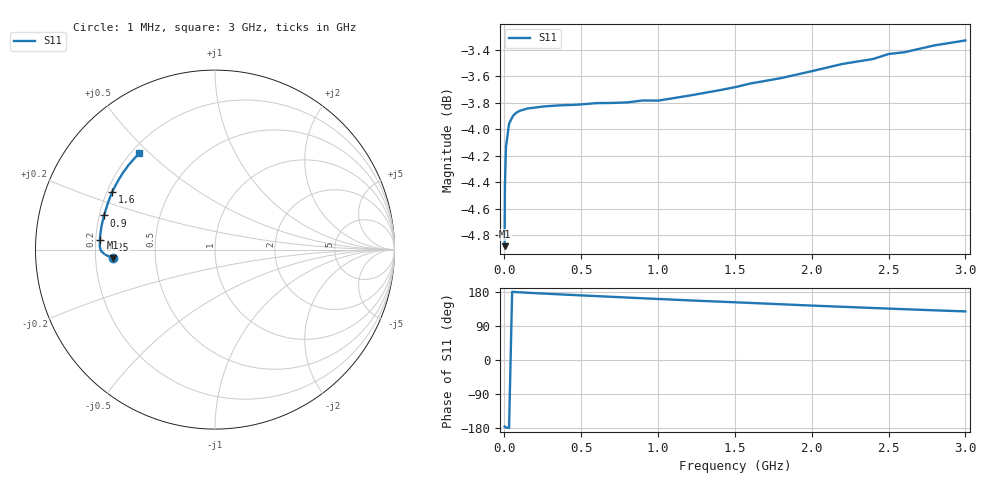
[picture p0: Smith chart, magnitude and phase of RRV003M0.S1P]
! SIEMENS Small Signal Semiconductors
! BA595
! Si PIN Diode in SOD323
! IF = 3 mA
! S-Parameters:  July  1992
# GHz  S  MA  R  50
!  f  S11
! GHz  MAG  ANG
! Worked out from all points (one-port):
!   33 points, 1 MHz to 3 GHz, reference 50 ohm
!   lowest |S11| = -4.9 dB at 1 MHz (marker M1), VSWR 3.65, Z = 13.7 - j1.82 ohm
!   |S11| at or under -10 dB: nowhere
!   S11 on the Smith chart (normalised r, x): 1 MHz: 0.27, -0.04; 250 MHz: 0.22, +0.04; 900 MHz: 0.22, +0.14; 1.6 GHz: 0.22, +0.25; 3 GHz: 0.23, +0.46
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0.001  0.5699 -175.5
0.003  0.6007 -176.7
0.01  0.6214 -178.1
0.03  0.634 -179.3
0.06  0.6388 179.7
0.08  0.6403 179.1
0.1  0.6412 178.7
0.15  0.6425 177.5
0.2  0.643 176.4
0.25  0.6436 175.4
0.4  0.6444 172.4
0.45  0.6445 171.5
0.5  0.6448 170.5
0.6  0.6455 168.6
0.8  0.6459 164.8
0.9  0.647 162.9
1  0.6469 161.1
1.2  0.6497 157.4
1.4  0.6528 154.0
1.6  0.6566 150.6
1.8  0.6597 147.1
2  0.6637 143.6
2.2  0.6679 140.4
2.4  0.6708 137.2
2.5  0.6737 135.7
2.6  0.6747 134.1
2.8  0.6788 131.1
3  0.6817 128.2
